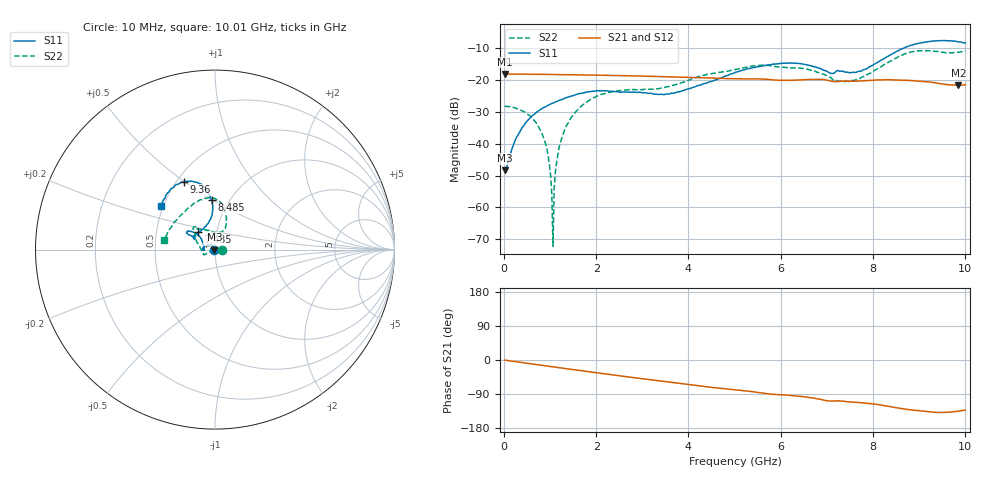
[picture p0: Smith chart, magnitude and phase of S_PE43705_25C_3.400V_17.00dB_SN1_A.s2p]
! Device ID: PE43705
! Serial: 1
! Insertion: A
! Impedance: 50 ohm
! Temp: 25C
! VDD: 3.400V
! Attenuation Step: 17.00dB
#  Hz  S  RI  R  50
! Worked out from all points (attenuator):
!   401 points, 10 MHz to 10.01 GHz, reference 50 ohm
!   highest |S21| = -18.04 dB at 10 MHz (marker M1); lowest = -21.6 dB at 9.86 GHz (marker M2)
!   lowest |S11| = -48.4 dB at 10 MHz (marker M3), VSWR 1.01, Z = 49.6 + j0.0446 ohm
!   |S11| at or under -10 dB: start of sweep to 8.659 GHz
!   |S22| runs from -72.2 to -10.7 dB; largest |S21 - S12| = 0.0014
!   S11 on the Smith chart (normalised r, x): 10 MHz: 0.99, +0.00; 7.435 GHz: 0.82, +0.16; 8.485 GHz: 0.83, +0.49; 9.36 GHz: 0.55, +0.50; 10.01 GHz: 0.49, +0.27
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1e7  -0.0038 0.000449  0.1254 -0.00055  0.1254 -0.00049  0.0389 -1.01e-06
3.35e8  -0.00616 0.0139  0.1238 -0.0129  0.1236 -0.0127  0.0344 0.00405
7.6e8  -0.0208 0.0261  0.1205 -0.028  0.1205 -0.0279  0.0169 0.00507
9.35e8  -0.0285 0.0274  0.1184 -0.0342  0.1186 -0.034  0.00741 0.00267
9.85e8  -0.0312 0.0274  0.1178 -0.0358  0.1179 -0.0358  0.00426 0.0015
1.01e9  -0.0323 0.0273  0.1175 -0.0367  0.1175 -0.0366  0.00297 0.000935
1.06e9  -0.0345 0.0272  0.1166 -0.0382  0.1167 -0.0382  -0.000198 0.000146
1.11e9  -0.0367 0.0267  0.1161 -0.0398  0.1161 -0.0397  -0.00329 -0.00129
1.16e9  -0.0389 0.0266  0.1154 -0.0414  0.1154 -0.0414  -0.00606 -0.00214
1.26e9  -0.043 0.0253  0.1139 -0.0447  0.114 -0.0446  -0.0121 -0.00449
1.685e9  -0.0599 0.0167  0.1064 -0.0576  0.1065 -0.0575  -0.0364 -0.016
2.285e9  -0.0669 -0.000104  0.0935 -0.0735  0.0937 -0.0734  -0.0576 -0.0284
3.36e9  -0.0595 0.00333  0.0652 -0.0937  0.0653 -0.0935  -0.0735 -0.0048
5.01e9  -0.1001 0.0862  0.0207 -0.1035  0.0209 -0.1035  -0.1139 0.0939
6.01e9  -0.1534 0.1011  -0.00296 -0.0995  -0.00246 -0.0994  -0.1039 0.1221
6.685e9  -0.1447 0.0817  -0.0182 -0.1012  -0.018 -0.1011  -0.084 0.1142
7.435e9  -0.0921 0.097  -0.033 -0.0909  -0.0327 -0.091  0.0122 0.096
8.36e9  -0.0125 0.2452  -0.0547 -0.0857  -0.0549 -0.0858  0.0622 0.1857
8.485e9  -0.0185 0.2754  -0.0584 -0.0824  -0.0584 -0.083  0.0564 0.2125
9.36e9  -0.1717 0.3773  -0.0678 -0.0606  -0.0674 -0.0609  -0.1034 0.2633
9.86e9  -0.2771 0.2875  -0.0587 -0.0587  -0.0587 -0.0584  -0.2461 0.1216
1.001e10  -0.3012 0.2405  -0.0574 -0.0626  -0.0578 -0.0629  -0.2853 0.0545
